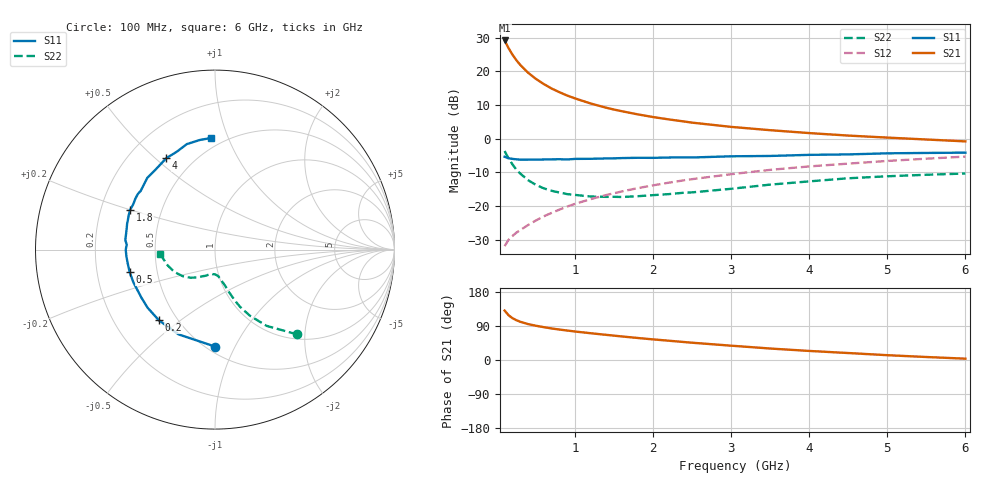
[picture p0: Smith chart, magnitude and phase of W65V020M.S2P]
! SIEMENS Small Signal Semiconductors
! BFR193W
! Si NPN RF Bipolar Junction Transistor in SOT323
! VCE = 5 V  IC = 20 mA
! Common Emitter S-Parameters:  September  1992
# GHz  S  MA  R  50
!  f  S11  S21  S12  S22
! GHz  MAG  ANG  MAG  ANG  MAG  ANG  MAG  ANG
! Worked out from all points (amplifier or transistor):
!   28 points, 100 MHz to 6 GHz, reference 50 ohm
!   highest |S21| = 29.2 dB at 100 MHz (marker M1)
!   |S21| within 3 dB of that: start of sweep to 169.1 MHz
!   unconditionally stable (mu >= 1): 769 MHz to 2.583 GHz
!   at 300 MHz: K = 0.76, MSG = 24.5 dB, |S12| = -27.1 dB
!   at 1.5 GHz: K = 1.04, MAG = 11.2 dB, |S12| = -16.2 dB
!   at 6 GHz: K = 0.90, MSG = 2.3 dB, |S12| = -5.3 dB
!   lowest NFmin = 1.40 dB at 450 MHz
!   S11 on the Smith chart (normalised r, x): 100 MHz: 0.55, -0.84; 200 MHz: 0.40, -0.42; 500 MHz: 0.35, -0.11; 1.8 GHz: 0.33, +0.20; 4 GHz: 0.36, +0.54; 6 GHz: 0.43, +0.87
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0.1  0.5404 -89.9  28.89 130.4  0.0254 59.1  0.6582 -45.9
0.15  0.5142 -113.3  22.26 118.3  0.0315 55.5  0.5131 -55.9
0.2  0.5028 -128.4  17.83 110.4  0.0359 55.0  0.4175 -62.1
0.25  0.4959 -139.2  14.74 105.1  0.0403 56.0  0.3492 -66.3
0.3  0.4898 -146.7  12.54 100.9  0.044 57.4  0.3048 -68.7
0.4  0.4899 -158.0  9.595 94.8  0.0523 60.2  0.2431 -72.2
0.5  0.4918 -165.2  7.769 90.4  0.0611 62.4  0.2069 -74.5
0.6  0.4924 -171.1  6.523 86.7  0.0704 64.2  0.184 -77.2
0.7  0.4949 -175.5  5.598 83.3  0.0791 65.5  0.1691 -78.8
0.8  0.4974 -179.9  4.933 80.4  0.0885 66.4  0.1593 -81.0
0.9  0.4927 176.8  4.396 77.8  0.0984 67.0  0.1508 -82.4
1  0.5025 173.9  3.988 75.2  0.1077 67.3  0.1467 -84.3
1.2  0.5044 168.0  3.348 70.7  0.1269 67.3  0.1389 -88.9
1.5  0.5124 161.4  2.719 64.3  0.1552 66.7  0.1375 -95.4
1.8  0.5222 155.1  2.311 58.2  0.1844 65.6  0.1402 -101.3
2.2  0.5271 147.2  1.942 50.9  0.2226 63.5  0.1506 -107.8
3  0.5495 133.4  1.503 37.8  0.2979 58.0  0.1808 -121.4
3.5  0.5559 126.3  1.342 30.3  0.3454 54.1  0.2086 -131.2
4  0.5772 118.0  1.216 23.9  0.3885 49.7  0.233 -140.6
4.5  0.5861 111.0  1.116 18.4  0.4278 45.7  0.2591 -151.4
5.5  0.6162 98.1  0.976 7.9  0.5063 37.4  0.2921 -169.5
6  0.6226 92.0  0.915 3.5  0.5437 32.9  0.3049 -175.1
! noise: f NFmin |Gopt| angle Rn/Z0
0.45  1.4  0.3  160  0.1
0.9  1.45  0.34  172  0.11
1.8  2.2  0.56  -148  0.2
